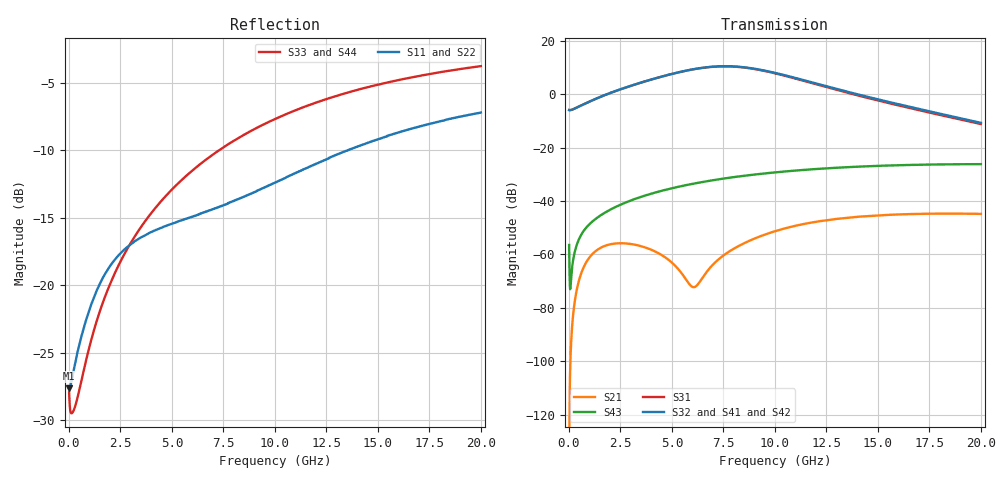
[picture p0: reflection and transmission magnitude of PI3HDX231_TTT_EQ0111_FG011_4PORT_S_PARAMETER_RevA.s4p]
! NPort=4 DATA=2000 NOISE=0 GROUPDELAY=0 COMPLEX_DATAFORMAT=POLAR
! NumOfBlock=1 NumOfParam=0
! .MODEL Smodel S TSTONEFILE=PI3HDX231_TTT_EQ0111_FG011_4PORT_S_PARAMETER_RevA.s4p TYPE=S
!  -- The above .MODEL line can be used for the S element in the netlist.
! The s parameter is extracted from the linear redriver, it is not bi-directional; only s(4,1)s(4,2) and s(3,1)s(3,2)
! should be the insertion loss
!Port definition:
!Port1 = input+
!Port2 = input-
!Port3 = output+
!Port4 = output-
# Hz S MA R  50
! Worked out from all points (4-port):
!   2000 points, 10 MHz to 20 GHz, reference 50 ohm
!   strongest paths, dB at 10 MHz, 5.01 GHz, 10.01 GHz, 15.01 GHz, 20 GHz:
!     S32: -5.9, 7.6, 8.0, -2.0, -10.7
!     S41: -5.9, 7.6, 8.0, -2.0, -10.9
!     S42: -5.9, 7.7, 7.9, -2.2, -10.9
!     S31: -5.9, 7.6, 7.8, -2.4, -11.2
!     S43: -56.5, -35.2, -29.3, -26.9, -26.2
!     S21: -134.8, -63.2, -51.3, -45.4, -44.8
!   lowest |S11| = -27.6 dB at 10 MHz (marker M1), VSWR 1.09, Z = 46 - j0.0776 ohm
!   |S11| at or under -10 dB: start of sweep to 13.55 GHz
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1e7  0.04152 -178.8  1.825e-07 -13.9  0 0.0  0 0.0
     1.825e-07 -14.0  0.04152 -178.8  0 0.0  0 0.0
     0.5042 -0.3  0.5042 179.7  0.04012 -3.2  0.0015 -70.3
     0.5042 179.7  0.5042 -0.3  0.0015 -70.3  0.04012 -3.2
4.79e9  0.1668 -140.3  0.0008143 -12.4  4.312e-10 -164.1  2.392e-10 -140.6
        0.0008165 -12.3  0.1668 -140.4  2.313e-10 -140.5  4.481e-10 -163.9
        2.278 -49.2  2.283 130.4  0.2176 -101.8  0.01657 62.7
        2.292 130.3  2.297 -48.4  0.01653 62.6  0.2176 -101.8
6.73e9  0.1881 -136.5  0.0004928 94.2  3.555e-09 133.2  1.751e-09 -174.5
        0.0004922 93.1  0.1878 -136.7  1.695e-09 -173.4  3.712e-09 132.4
        3.185 -108.1  3.202 71.7  0.2945 -107.4  0.0236 51.5
        3.211 71.4  3.218 -107.2  0.02352 51.5  0.2946 -107.4
8.49e9  0.2124 -132.4  0.001617 96.5  1.294e-08 77.1  8.614e-09 140.1
        0.001606 96.0  0.2117 -132.6  8.414e-09 141.7  1.347e-08 75.4
        3.154 -169.6  3.193 10.1  0.36 -112.0  0.02967 40.3
        3.198 9.7  3.191 -168.6  0.02955 40.4  0.3602 -112.0
1.084e10  0.257 -128.7  0.003342 75.4  4.071e-08 15.0  3.449e-08 66.7
          0.00332 75.1  0.2555 -128.8  3.409e-08 68.5  4.168e-08 12.6
          2.032 119.0  2.085 -61.5  0.4391 -117.6  0.03677 25.0
          2.083 -62.1  2.06 120.2  0.03664 25.2  0.4392 -117.7
1.383e10  0.322 -128.6  0.005018 44.8  1.132e-07 -49.8  9.471e-08 -13.0
          0.00498 44.5  0.32 -128.5  9.481e-08 -11.3  1.14e-07 -52.3
          0.9901 54.7  1.034 -127.0  0.5235 -124.2  0.04359 5.5
          1.028 -127.6  1.009 56.2  0.04352 5.8  0.5234 -124.2
2e10  0.4355 -135.6  0.005777 -4.4  3.683e-07 -159.6  2.745e-07 -135.7
      0.005729 -4.5  0.4338 -135.4  2.78e-07 -134.7  3.642e-07 -161.6
      0.2752 -41.9  0.2903 132.4  0.6464 -135.0  0.04882 -32.3
      0.2863 132.2  0.2846 -40.4  0.04893 -32.0  0.6461 -135.0
